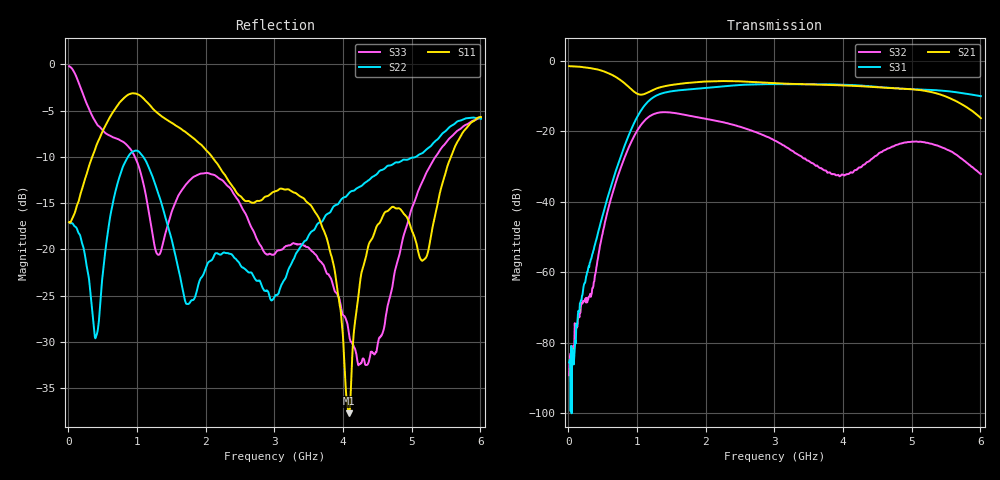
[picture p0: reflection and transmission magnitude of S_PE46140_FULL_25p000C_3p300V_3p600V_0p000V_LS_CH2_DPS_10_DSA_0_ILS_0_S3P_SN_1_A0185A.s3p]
! Device ID: PE46140_FULL
! File Path: z:\PE46140\MajorStates\25p000C\3p300\LS_CH2_DPS_10_DSA_0_ILS_0\PE46140_FULL_25p000C_3p300V_3p600V_0p000V_LS_CH2_DPS_10_DSA_0_ILS_0_S3P_SN_1_A0185A.s3p
! Serial: 1
! Lot: A0185A
! Temp: 25.000C
! VDD: 3.300
! VSS: 0.000
! Control_Hi: 3.600
! Control_Lo: 0.000
! Logic State: LS_CH2_DPS_10_DSA_0_ILS_0
! Port 1: RFIN
! Port 2: RFOUT1
! Port 3: RFOUT2
! ThroughPath:1-3
! IDD: 0.0003147783
! ISS: -1.046e-007
! Comment:
#  Hz  S  RI  R  50
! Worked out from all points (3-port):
!   801 points, 10 MHz to 6.01 GHz, reference 50 ohm
!   strongest paths, dB at 10 MHz, 1.51 GHz, 3.01 GHz, 4.51 GHz, 6.01 GHz:
!     S21: -1.5, -6.8, -6.3, -7.5, -16.3
!     S31: -85.6, -8.6, -6.6, -7.4, -10.0
!     S32: -89.2, -14.7, -22.7, -26.5, -32.1
!   lowest |S11| = -37.7 dB at 4.09 GHz (marker M1), VSWR 1.03, Z = 50.7 - j1.12 ohm
!   |S11| at or under -10 dB: start of sweep to 346.2 MHz; 2.094 GHz to 5.574 GHz (3.48 GHz wide, 90.8 % of centre)
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1e7  0.1401 -0.0109  0.8419 -0.0244  1.84e-05 -6.1e-06
     0.8419 -0.0244  0.14 -0.00677  6.99e-06 -3.35e-06
     -2.84e-05 4.43e-05  3.42e-05 4.77e-06  0.9746 -0.0928
1.45e8  0.1152 -0.1393  0.7687 -0.3091  0.000135 -0.000214
        0.7685 -0.3094  0.1068 -0.0617  -0.000161 0.000142
        0.000158 -0.000235  -0.000158 0.000176  0.2548 -0.7639
3.55e8  -0.016 -0.3218  0.4591 -0.6282  -0.000314 -0.0019
        0.4593 -0.6262  -0.00909 -0.0426  -0.000595 5.44e-06
        -0.000361 -0.00183  -0.000596 -2.11e-05  -0.4628 -0.2358
7.075e8  -0.4709 -0.3661  -0.1595 -0.555  -0.0213 -0.0223
         -0.1587 -0.5557  0.1019 0.1971  -0.0206 0.00551
         -0.0212 -0.0223  -0.0205 0.0055  -0.0558 0.3936
1.12e9  -0.6106 0.1869  -0.1898 -0.2845  -0.1167 0.2088
        -0.1899 -0.2853  0.2528 -0.17  0.131 0.0637
        -0.1172 0.2089  0.1309 0.064  0.1525 -0.1354
1.6825e9  -0.2777 0.3378  -0.4793 -0.0419  0.3777 -0.0894
          -0.4796 -0.0422  0.0253 -0.0506  -0.1569 -0.0716
          0.3781 -0.0894  -0.157 -0.0716  0.0949 0.195
3.01e9  -0.0282 0.2039  0.4067 0.2592  -0.4536 0.1153
        0.4062 0.2603  -0.0558 -0.000271  0.0229 -0.0701
        -0.4539 0.1151  0.023 -0.07  0.0942 -0.0111
4.09e9  0.0069 -0.011  -0.00696 -0.4445  0.3403 0.3054
        -0.00666 -0.445  0.1535 0.1318  0.0222 -0.0118
        0.3406 0.3051  0.0222 -0.0118  0.0253 -0.0237
4.4875e9  -0.1102 -0.0734  -0.3202 -0.2753  0.4277 -0.0173
          -0.3204 -0.2759  0.2415 0.079  -0.0368 -0.0264
          0.428 -0.0174  -0.0367 -0.0263  0.0265 0.00847
6.01e9  -0.4358 -0.2839  0.1488 0.0379  -0.3069 -0.0712
        0.149 0.0381  0.248 -0.4434  0.00322 -0.0244
        -0.308 -0.0705  0.00309 -0.0246  0.506 -0.1069
